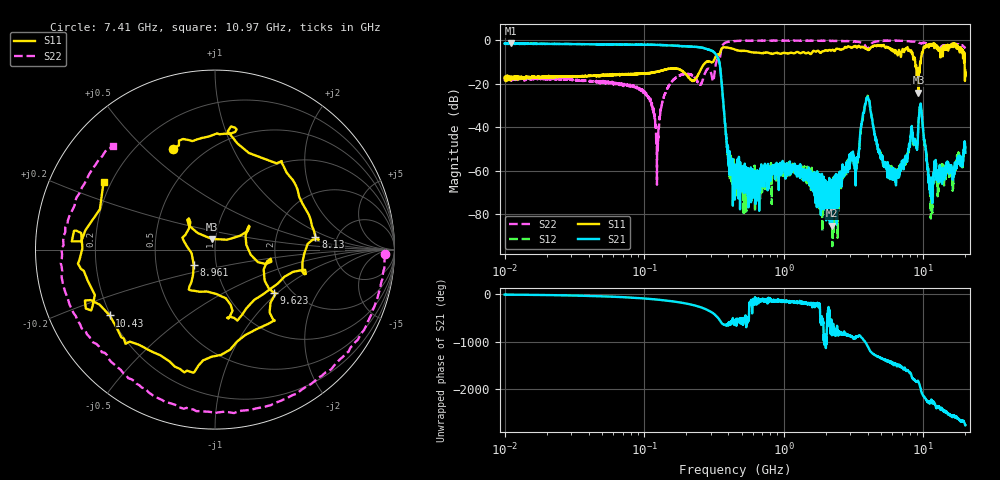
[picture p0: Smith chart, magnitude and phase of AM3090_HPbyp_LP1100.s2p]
# Hz S DB R 50
!freq MagS11 AngS11 MagS21 AngS21 MagS12 AngS12 MagS22 AngS22
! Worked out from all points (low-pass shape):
!   3201 points, 10 MHz to 20 GHz, reference 50 ohm
!   highest |S21| = -1.42 dB at 11.1 MHz (marker M1); lowest = -85.3 dB at 2.222 GHz (marker M2)
!   |S21| within 3 dB of the highest: start of sweep to 288.9 MHz; 289 MHz to 290.5 MHz (1.453 MHz wide, 0.501 % of centre)
!   lowest |S11| = -24.2 dB at 9.22 GHz (marker M3), VSWR 1.13, Z = 48 + j5.7 ohm
!   |S11| at or under -10 dB: start of sweep to 278.5 MHz; 8.732 GHz to 9.483 GHz (750.9 MHz wide, 8.24 % of centre); 19.73 GHz to end of sweep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
!   |S22| runs from -66.5 to -0.2 dB; largest |S21 - S12| = 0.044
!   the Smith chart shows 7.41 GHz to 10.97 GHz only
!   S11 on the Smith chart (normalised r, x): 7.41 GHz: 0.34, +0.61; 8.13 GHz: 3.43, +0.72; 8.961 GHz: 0.78, -0.13; 9.623 GHz: 1.64, -0.94; 10.43 GHz: 0.20, -0.28; 10.97 GHz: 0.17, +0.27
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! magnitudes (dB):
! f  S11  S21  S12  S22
! 10 MHz  -17.5  -1.6  -1.5  -17.6
! 11.1 MHz  -17.9  -1.4  -1.9  -17.5
! 35.55 MHz  -16.6  -1.9  -1.8  -18.5
! 97.1 MHz  -15.5  -2.1  -2.1  -23.4
! 126.1 MHz  -14.5  -2.2  -2.2  -46.7
! 157.6 MHz  -13.0  -2.5  -2.5  -19.1
! 329.2 MHz  -6.9  -7.0  -7.0  -9.8
! 400 MHz  -3.5  -51.8  -52.7  -0.8
! 447.2 MHz  -4.3  -63.0  -59.4  -0.5
! 1.59 GHz  -5.8  -61.1  -62.3  -0.3
! 2.222 GHz  -4.5  -85.3  -84.0  -0.4
! 3.32 GHz  -3.3  -53.9  -57.5  -0.6
! 3.968 GHz  -4.4  -26.9  -25.8  -4.1
! 5.639 GHz  -3.6  -59.4  -59.9  -0.3
! 7.41 GHz  -4.3  -54.8  -54.9  -0.5
! 8.13 GHz  -5.0  -43.6  -44.9  -0.6
! 8.961 GHz  -16.8  -48.8  -49.3  -0.9
! 9.22 GHz  -24.2  -38.8  -38.9  -1.1
! 9.623 GHz  -7.9  -30.5  -30.5  -1.5
! 10.43 GHz  -3.2  -50.8  -51.1  -1.5
! 10.97 GHz  -2.8  -66.0  -63.7  -1.8
! 20 GHz  -14.0  -51.8  -50.0  -3.8
